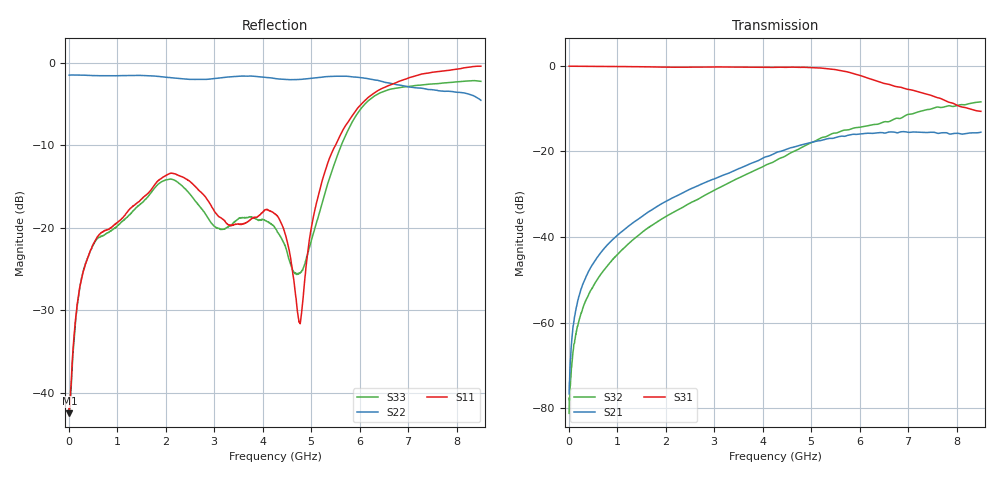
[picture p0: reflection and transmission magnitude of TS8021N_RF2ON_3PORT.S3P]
!Agilent Technologies,E5071C,MY46522130,B.12.04
!Date: Mon Jun 30 18:15:14 2025
!Data & Calibration Information:
!Freq	S11:SOLT4(ON)	S12:SOLT4(ON)	S13:SOLT4(ON)
!	S21:SOLT4(ON)	S22:SOLT4(ON)	S23:SOLT4(ON)
!	S31:SOLT4(ON)	S32:SOLT4(ON)	S33:SOLT4(ON)
!PortZ  Port1:50+j0  Port2:50+j0  Port3:50+j0
!Above PortZ is port z conversion or system Z0 setting when saving the data.
!When reading, reference impedance value at option line is always used.
# Hz S dB R 50
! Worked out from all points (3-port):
!   1601 points, 10 MHz to 8.5 GHz, reference 50 ohm
!   strongest paths, dB at 10 MHz, 2.132 GHz, 4.255 GHz, 6.378 GHz, 8.5 GHz:
!     S31: -0.1, -0.4, -0.4, -3.6, -10.7
!     S21: -76.6, -30.9, -20.4, -15.7, -15.5
!     S32: -81.1, -34.4, -22.2, -13.6, -8.4
!   lowest |S11| = -42.5 dB at 15.31 MHz (marker M1), VSWR 1.02, Z = 50.7 - j0.228 ohm
!   |S11| at or under -10 dB: start of sweep to 5.504 GHz
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1e7  -41.91 -5.5  -77.46 56.7  -0.12 -0.2
     -76.59 46.4  -1.52 179.8  -80.10 36.7
     -0.12 -0.2  -81.14 26.6  -42.00 -5.2
1.530625e7  -42.49 -17.4  -74.25 55.6  -0.12 -0.3
            -73.98 58.2  -1.51 179.7  -77.64 44.0
            -0.12 -0.3  -77.48 46.3  -42.48 -14.7
2.275562e8  -27.27 -86.7  -53.26 88.8  -0.13 -4.4
            -53.26 89.1  -1.51 177.0  -59.00 91.0
            -0.13 -4.5  -58.96 91.5  -27.33 -86.7
7.794062e8  -20.28 -104.6  -42.06 93.8  -0.19 -15.0
            -42.07 93.9  -1.59 168.2  -47.03 103.5
            -0.18 -15.0  -46.92 103.0  -20.71 -100.3
2.095356e9  -13.43 -105.1  -31.15 92.0  -0.35 -39.7
            -31.14 92.0  -1.82 146.3  -34.60 102.5
            -0.36 -39.7  -34.63 102.3  -14.12 -147.8
4.255e9  -18.33 -119.0  -20.62 63.8  -0.34 -85.1
         -20.42 64.2  -1.92 104.9  -21.98 80.7
         -0.37 -85.0  -22.25 81.4  -20.02 142.6
4.7644e9  -31.53 149.6  -18.74 50.2  -0.37 -98.2
          -18.60 51.0  -2.04 92.1  -19.13 72.3
          -0.39 -98.2  -19.34 71.9  -25.51 -156.3
5.210125e9  -14.70 79.7  -17.29 37.7  -0.58 -112.0
            -17.44 38.9  -1.78 83.7  -16.87 59.9
            -0.56 -111.8  -16.83 58.5  -17.35 -143.7
5.915856e9  -5.84 86.7  -15.95 17.0  -1.97 -136.0
            -16.02 16.9  -1.75 86.0  -14.53 34.4
            -1.99 -135.6  -14.46 34.3  -6.50 166.6
8.5e9  -0.43 60.2  -15.67 -36.5  -10.62 -169.2
       -15.52 -35.3  -4.56 47.4  -8.19 -32.8
       -10.66 -170.8  -8.44 -34.1  -2.26 112.1
